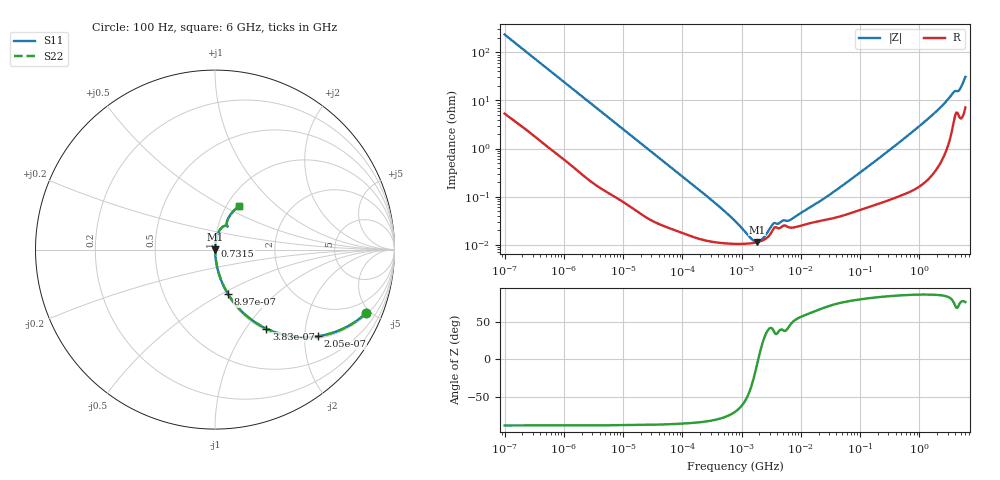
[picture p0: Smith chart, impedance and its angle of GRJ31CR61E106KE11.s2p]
!Murata Part Number: GRJ31CR61E106KE11
!These Parameters are Measured in Series Mode Connection
!Data Generated on Jun 19, 2026
!  o--ll--o
!Port1  Port2
!  o------o
!Operation Temp=25[degC], DC Bias Voltage=0[V]
!Freq. Start=100[Hz] Stop=6[GHz] 401[Steps]
# Hz S RI R 50
!Freq.(Hz) S11(Real) S11(Imag) S21(Real) S21(Imag) S12(Real) S12(Imag) S22(Real) S22(Imag)
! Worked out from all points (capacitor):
!   401 points, 100 Hz to 6 GHz, reference 50 ohm
!   read as one part in series: C = 6.74 uF near 109 Hz
!   lowest |Z| = 11.4 mohm at 1.814 MHz (marker M1)
!   series resonance near 1.912 MHz, so ESL is about 1 nH
!   S11 on the Smith chart (normalised r, x): 100 Hz: 1.11, -4.70; 205 Hz: 1.06, -2.32; 383 Hz: 1.03, -1.25; 897 Hz: 1.01, -0.54; 731.5 MHz: 1.00, +0.04; 6 GHz: 1.14, +0.60
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100  0.8412 -0.3543  0.1588 0.3543  0.1588 0.3543  0.8412 -0.3543
205  0.5722 -0.483  0.4278 0.483  0.4278 0.483  0.5722 -0.483
383  0.2863 -0.4402  0.7137 0.4402  0.7137 0.4402  0.2863 -0.4402
897  0.0736 -0.2493  0.9264 0.2493  0.9264 0.2493  0.0736 -0.2493
2008  0.0176 -0.12  0.9824 0.12  0.9824 0.12  0.0176 -0.12
6433  0.00258 -0.0387  0.9974 0.0387  0.9974 0.0387  0.00258 -0.0387
40335  0.000309 -0.00638  0.9997 0.00638  0.9997 0.00638  0.000309 -0.00638
302498  0.000117 -0.000865  0.9999 0.000865  0.9999 0.000865  0.000117 -0.000865
774597  0.000104 -0.000294  0.9999 0.000294  0.9999 0.000294  0.000104 -0.000294
1449809  0.000107 -8.11e-05  0.9999 8.11e-05  0.9999 8.11e-05  0.000107 -8.11e-05
1813585  0.000112 -1.54e-05  0.9999 1.54e-05  0.9999 1.54e-05  0.000112 -1.54e-05
2268635  0.000123 5.11e-05  0.9999 -5.11e-05  0.9999 -5.11e-05  0.000123 5.11e-05
3549919  0.000226 0.000169  0.9998 -0.000169  0.9998 -0.000169  0.000226 0.000169
6644369  0.000226 0.000239  0.9998 -0.000239  0.9998 -0.000239  0.000226 0.000239
1.555665e7  0.000288 0.000566  0.9997 -0.000566  0.9997 -0.000566  0.000288 0.000566
4.556224e7  0.000388 0.0015  0.9996 -0.0015  0.9996 -0.0015  0.000388 0.0015
3.124326e8  0.000933 0.00918  0.9991 -0.00918  0.9991 -0.00918  0.000933 0.00918
7.31507e8  0.00174 0.0211  0.9983 -0.0211  0.9983 -0.0211  0.00174 0.0211
1.95892e9  0.00722 0.0591  0.9928 -0.0591  0.9928 -0.0591  0.00722 0.0591
3.666503e9  0.0442 0.128  0.9558 -0.128  0.9558 -0.128  0.0442 0.128
4.586474e9  0.0661 0.1329  0.9339 -0.1329  0.9339 -0.1329  0.0661 0.1329
6e9  0.1349 0.243  0.8651 -0.243  0.8651 -0.243  0.1349 0.243
